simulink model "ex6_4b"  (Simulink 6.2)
settings: Solver=ode45  SolverMode=SingleTasking  StartTime=0.0  StopTime=10.0  MaxStep=1  RelTol=1e-3  AbsTol=1e-6

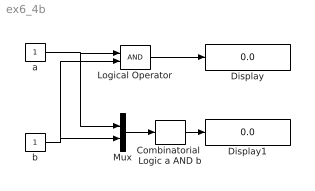
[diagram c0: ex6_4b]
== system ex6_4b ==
  Combinatorial  Logic a AND b : CombinatorialLogic  TruthTable=[0;0;0;1]
  Display : Display
  Display1 : Display
  Logical Operator : Logic
  Mux : Mux  Inputs=2
  a : Constant
  b : Constant
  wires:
  b/1 -> Logical Operator/2, Mux/2
  Mux/1 -> Combinatorial  Logic a AND b/1
  Combinatorial  Logic a AND b/1 -> Display1/1
  Logical Operator/1 -> Display/1
  a/1 -> Logical Operator/1, Mux/1
